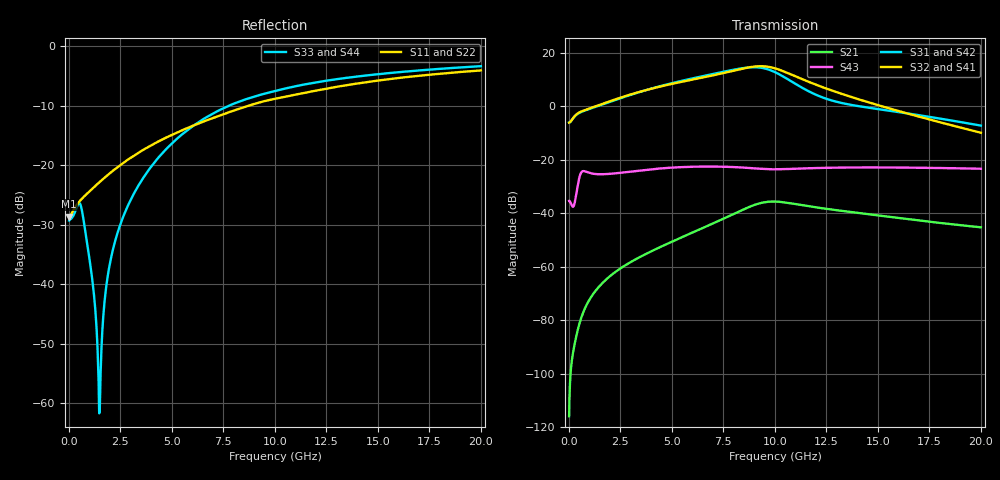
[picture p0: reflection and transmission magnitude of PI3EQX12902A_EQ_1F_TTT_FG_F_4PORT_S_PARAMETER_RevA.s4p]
! NPort=4 DATA=2000 NOISE=0 GROUPDELAY=0 COMPLEX_DATAFORMAT=POLAR
! NumOfBlock=1 NumOfParam=0
! .MODEL Smodel S TSTONEFILE=PI3EQX12902A_EQ_1F_TTT_FG_F_4PORT_S_PARAMETER_RevA.s4p TYPE=S
!  -- The above .MODEL line can be used for the S element in the netlist.
! The s parameter is extracted from the linear redriver, it is not bi-directional; only s(4,1)s(4,2) and s(3,1)s(3,2)
! should be the insertion loss
!Port definition:
!Port1 = input+
!Port2 = input-
!Port3 = output+
!Port4 = output-
# Hz S MA R  50
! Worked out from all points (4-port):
!   2000 points, 10 MHz to 20 GHz, reference 50 ohm
!   strongest paths, dB at 10 MHz, 5.01 GHz, 10.01 GHz, 15.01 GHz, 20 GHz:
!     S32: -6.0, 8.5, 14.3, 0.5, -9.8
!     S41: -6.0, 8.5, 14.2, 0.5, -9.8
!     S31: -6.0, 8.7, 12.8, -1.0, -7.2
!     S42: -6.0, 8.7, 12.7, -1.2, -7.3
!     S43: -35.3, -22.9, -23.5, -22.8, -23.3
!     S21: -116.0, -50.6, -35.6, -40.8, -45.2
!   lowest |S11| = -28.6 dB at 10 MHz (marker M1), VSWR 1.08, Z = 46.4 - j0.0607 ohm
!   |S11| at or under -10 dB: start of sweep to 8.722 GHz
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1e7  0.03704 -179.0  1.589e-06 51.9  0 0.0  0 0.0
     1.589e-06 51.9  0.03704 -179.0  0 0.0  0 0.0
     0.4991 1.2  0.4991 -178.8  0.03429 6.0  0.01709 -177.1
     0.4991 -178.8  0.4991 1.2  0.01709 -177.1  0.03429 6.0
5.84e9  0.2086 -111.9  0.004101 100.9  1.438e-06 -19.0  9.048e-07 88.5
        0.004102 100.9  0.2086 -111.9  9.077e-07 88.7  1.432e-06 -18.8
        3.25 -51.3  3.099 110.7  0.2024 -44.8  0.07377 146.5
        3.089 110.6  3.213 -51.8  0.07415 146.6  0.2018 -44.8
8.03e9  0.289 -111.6  0.009851 76.9  7.464e-06 -82.9  4.529e-06 42.2
        0.00985 76.9  0.289 -111.7  4.554e-06 42.2  7.436e-06 -82.6
        4.904 -110.7  4.717 51.2  0.3302 -66.4  0.07282 123.4
        4.692 51.1  4.832 -111.1  0.07327 123.3  0.3295 -66.3
9.29e9  0.3382 -113.6  0.01551 44.9  1.388e-05 -131.4  1.109e-05 -3.0
        0.01549 44.9  0.3382 -113.6  1.113e-05 -3.2  1.382e-05 -131.0
        5.345 -163.0  5.685 -0.3  0.3902 -76.6  0.06772 113.5
        5.639 -0.4  5.261 -163.4  0.0681 113.4  0.3899 -76.5
1.043e10  0.3742 -115.9  0.01612 8.6  1.535e-05 -170.7  1.642e-05 -55.8
          0.01609 8.6  0.3742 -115.9  1.642e-05 -56.1  1.532e-05 -170.0
          3.593 148.2  4.541 -52.7  0.4378 -83.9  0.06678 109.4
          4.493 -52.6  3.529 147.7  0.06706 109.1  0.4377 -83.8
1.242e10  0.4367 -118.6  0.01227 -26.3  1.85e-05 160.9  1.894e-05 -121.2
          0.01225 -26.2  0.4368 -118.6  1.886e-05 -121.3  1.858e-05 161.6
          1.428 116.4  2.221 -109.3  0.5103 -94.8  0.07094 96.7
          2.198 -108.8  1.389 116.1  0.07097 96.4  0.5106 -94.7
2e10  0.6255 -131.7  0.005442 -76.9  3.944e-05 51.1  1.797e-05 95.2
      0.00547 -76.8  0.6255 -131.7  1.781e-05 95.7  3.977e-05 51.3
      0.4388 35.6  0.3219 128.6  0.6793 -119.6  0.0684 46.2
      0.3233 129.3  0.4324 36.3  0.06832 46.1  0.6797 -119.6
